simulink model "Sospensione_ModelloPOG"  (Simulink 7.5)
settings: Solver=ode45  StartTime=0.0  StopTime=10.0  MaxStep=1e-2  RelTol=1e-3
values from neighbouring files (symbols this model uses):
  b1 = 1000    [Exercises03.m]
  b2 = 10000    [Exercises03.m]
  g = 9.81    [Exercises03.m]
  K = 20000    [Exercises03.m]
  Kp = 190000    [Exercises03.m]
  Ma = 290    [Exercises03.m]
  Mr = 60    [Exercises03.m]
  x10 = 0    [Exercises03.m]
  x20 = 0    [Exercises03.m]
  x30 = 0    [Exercises03.m]
  x40 = 0    [Exercises03.m]

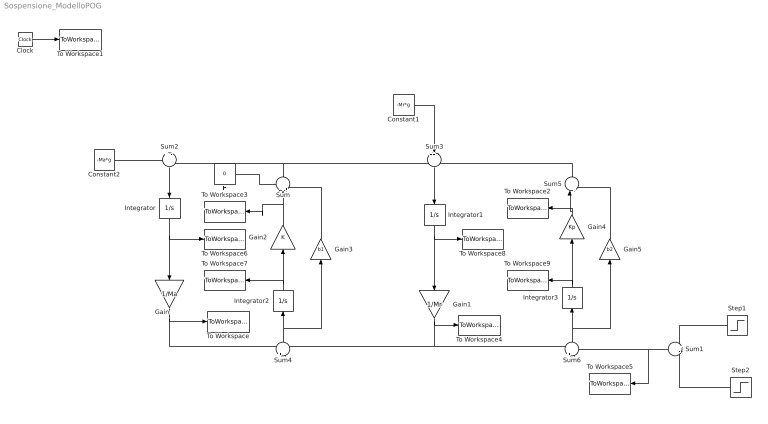
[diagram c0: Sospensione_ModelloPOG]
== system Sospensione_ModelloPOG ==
  Clock : Clock
  Constant1 : Constant  Value=-Mr*g  OutDataType=sfix(16)  OutScaling=2^0
  Constant2 : Constant  Value=-Ma*g  OutDataType=sfix(16)  OutScaling=2^0
  F : Constant  Value=0  OutDataType=sfix(16)  OutScaling=2^0
  Gain : Gain  Gain=1/Ma  ParameterDataType=sfix(16)  ParameterScaling=2^0  OutDataType=sfix(16)  OutScaling=2^0
  Gain1 : Gain  Gain=1/Mr  ParameterDataType=sfix(16)  ParameterScaling=2^0  OutDataType=sfix(16)  OutScaling=2^0
  Gain2 : Gain  Gain=K  ParameterDataType=sfix(16)  ParameterScaling=2^0  OutDataType=sfix(16)  OutScaling=2^0
  Gain3 : Gain  Gain=b1  ParameterDataType=sfix(16)  ParameterScaling=2^0  OutDataType=sfix(16)  OutScaling=2^0
  Gain4 : Gain  Gain=Kp  ParameterDataType=sfix(16)  ParameterScaling=2^0  OutDataType=sfix(16)  OutScaling=2^0
  Gain5 : Gain  Gain=b2  ParameterDataType=sfix(16)  ParameterScaling=2^0  OutDataType=sfix(16)  OutScaling=2^0
  Integrator : Integrator  InitialCondition=x10
  Integrator1 : Integrator  InitialCondition=x30
  Integrator2 : Integrator  InitialCondition=x20
  Integrator3 : Integrator  InitialCondition=x40
  Step1 : Step  Time=5  SampleTime=0
  Step2 : Step  Time=5+0.2  SampleTime=0
  Sum : Sum  Inputs=-++  OutDataType=sfix(16)  OutScaling=2^0
  Sum{1..2,4,6} (4 alike) : Sum  Inputs=+-  OutDataType=sfix(16)  OutScaling=2^0
  Sum3 : Sum  Inputs=++-  OutDataType=sfix(16)  OutScaling=2^0
  Sum5 : Sum  Inputs=|++  OutDataType=sfix(16)  OutScaling=2^0
  To Workspace : ToWorkspace  VariableName=dXma  SampleTime=-1  SaveFormat=Array
  To Workspace1 : ToWorkspace  VariableName=time  SampleTime=-1  SaveFormat=Array
  To Workspace2 : ToWorkspace  VariableName=Fp  SampleTime=-1  SaveFormat=Array
  To Workspace3 : ToWorkspace  VariableName=Fk  SampleTime=-1  SaveFormat=Array
  To Workspace4 : ToWorkspace  VariableName=dXmr  SampleTime=-1  SaveFormat=Array
  To Workspace5 : ToWorkspace  VariableName=dXs  SampleTime=-1  SaveFormat=Array
  To Workspace6 : ToWorkspace  VariableName=pa  SampleTime=-1  SaveFormat=Array
  To Workspace7 : ToWorkspace  VariableName=Xr  SampleTime=-1  SaveFormat=Array
  To Workspace8 : ToWorkspace  VariableName=pr  SampleTime=-1  SaveFormat=Array
  To Workspace9 : ToWorkspace  VariableName=Xrp  SampleTime=-1  SaveFormat=Array
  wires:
  Step1/1 -> Sum1/1
  Step2/1 -> Sum1/2
  Clock/1 -> To Workspace1/1
  Integrator/1 -> Gain/1, To Workspace6/1
  Sum2/1 -> Integrator/1
  Sum/1 -> Sum2/2, Sum3/1
  Gain2/1 -> Sum/2, To Workspace3/1
  Gain3/1 -> Sum/3
  Integrator2/1 -> To Workspace7/1, Gain2/1
  Gain/1 -> Sum4/1, To Workspace/1
  Sum4/1 -> Integrator2/1, Gain3/1
  Gain1/1 -> Sum4/2, Sum6/1, To Workspace4/1
  Integrator1/1 -> Gain1/1, To Workspace8/1
  Sum3/1 -> Integrator1/1
  Integrator3/1 -> Gain4/1, To Workspace9/1
  Sum6/1 -> Gain5/1, Integrator3/1
  Gain4/1 -> Sum5/1, To Workspace2/1
  Gain5/1 -> Sum5/2
  Sum5/1 -> Sum3/3
  F/1 -> Sum/1
  Constant2/1 -> Sum2/1
  Constant1/1 -> Sum3/2
  Sum1/1 -> Sum6/2, To Workspace5/1
